FUNCTION "KLASCHKA" : VOID
TITLE =SEQUENZA DOPPIO FOGLIO
AUTHOR : D_T
VERSION : 0.1

BEGIN
NETWORK
TITLE =Pulitura segnale 0 fogli da Klascka
//20131115_Reset o Fogli solo in Ciclo e Posizione di Prelievo
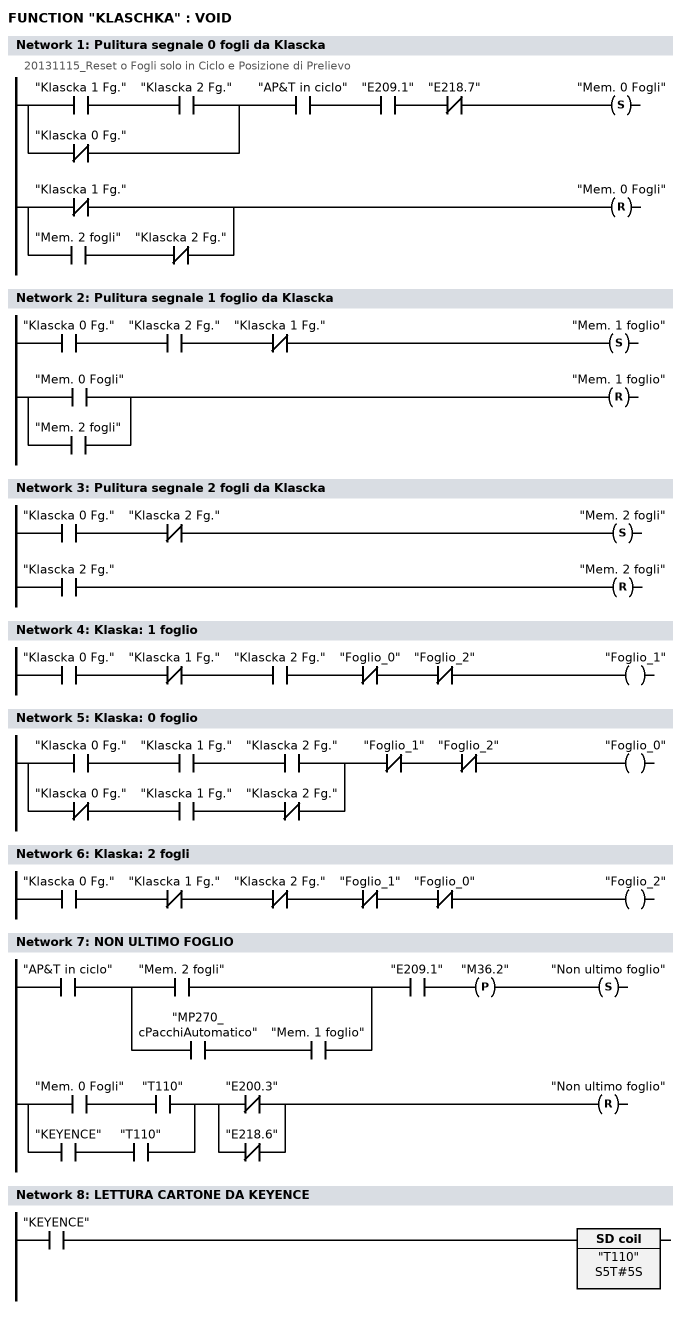
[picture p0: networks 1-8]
      U(    ;
      U     "Klascka 1 Fg.";
      U     "Klascka 2 Fg.";
      ON    "Klascka 0 Fg.";
      )     ;
      U     "AP&T  in ciclo";
      U     "E209.1";
      UN    "E218.7";
      S     "Mem. 0 Fogli";
      U(    ;
      ON    "Klascka 1 Fg.";
      O     ;
      U     "Mem. 2 fogli";
      UN    "Klascka 2 Fg.";
      )     ;
      R     "Mem. 0 Fogli";
      NOP   0;
NETWORK
TITLE =Pulitura segnale 1 foglio da Klascka

      U     "Klascka 0 Fg.";
      U     "Klascka 2 Fg.";
      UN    "Klascka 1 Fg.";
      S     "Mem. 1 foglio";
      U(    ;
      O     "Mem. 0 Fogli";
      O     "Mem. 2 fogli";
      )     ;
      R     "Mem. 1 foglio";
      NOP   0;
NETWORK
TITLE =Pulitura segnale 2 fogli da Klascka

      U     "Klascka 0 Fg.";
      UN    "Klascka 2 Fg.";
      S     "Mem. 2 fogli";
      U     "Klascka 2 Fg.";
      R     "Mem. 2 fogli";
      NOP   0;
NETWORK
TITLE =Klaska: 1 foglio

      U     "Klascka 0 Fg.";
      UN    "Klascka 1 Fg.";
      U     "Klascka 2 Fg.";
      UN    "Foglio_0";
      UN    "Foglio_2";
      =     "Foglio_1";
NETWORK
TITLE =Klaska: 0 foglio

      U(    ;
      U     "Klascka 0 Fg.";
      U     "Klascka 1 Fg.";
      U     "Klascka 2 Fg.";
      O     ;
      UN    "Klascka 0 Fg.";
      U     "Klascka 1 Fg.";
      UN    "Klascka 2 Fg.";
      )     ;
      UN    "Foglio_1";
      UN    "Foglio_2";
      =     "Foglio_0";
NETWORK
TITLE =Klaska: 2 fogli

      U     "Klascka 0 Fg.";
      UN    "Klascka 1 Fg.";
      UN    "Klascka 2 Fg.";
      UN    "Foglio_1";
      UN    "Foglio_0";
      =     "Foglio_2";
NETWORK
TITLE =NON ULTIMO FOGLIO

      U     "AP&T  in ciclo";
      U(    ;
      O     "Mem. 2 fogli";
      O     ;
      U     "MP270_cPacchiAutomatico";
      U     "Mem. 1 foglio";
      )     ;
      U     "E209.1";
      FP    "M36.2";
      S     "Non ultimo foglio";
      U(    ;
      U     "Mem. 0 Fogli";
      U     "T110";
      O     ;
      U     "KEYENCE";
      U     "T110";
      )     ;
      U(    ;
      ON    "E200.3";
      ON    "E218.6";
      )     ;
      R     "Non ultimo foglio";
      NOP   0;
NETWORK
TITLE =LETTURA CARTONE DA KEYENCE

      U     "KEYENCE";
      L     S5T#5S;
      SE    "T110";
      NOP   0;
      NOP   0;
      NOP   0;
      NOP   0;
NETWORK
TITLE =ULTIMO FOGLIO PRELEVATO
//A82.6  VECCHIO SEGNALE ORA NON ESISTE PIU'  PERCHE''?
//MaxZub20101019: T42 da 50MS a 150MS
      U(    ;
      U     "AP&T  in ciclo";
      U     "E209.1";
      U(    ;
      UN    "MP270_cPacchiAutomatico";
      U     "Mem. 1 foglio";
      O     ;
      UN    "Da Comau: Rich.svuotam.";
      UN    "M183.1";
      U     "MP270_cPacchiAutomatico";
      U(    ;
      U     "Mem. 0 Fogli";
      U     "T110";
      O     "T110";
      )     ;
      )     ;
      UN    "Non ultimo foglio";
      L     S5T#500MS;
      SE    "T42";
      NOP   0;
      NOP   0;
      NOP   0;
      U     "T42";
      )     ;
      FP    "One_Shot_ult_foglio";
      S     "Ultimo foglio prelevato";
      U(    ;
      O     "Cambio pacco in corso";
      O     "Non ultimo foglio";
      O(    ;
      U     "E209.1";
      FP    "One_R_Shot_ult_foglio";
      )     ;
      )     ;
      R     "Ultimo foglio prelevato";
      NOP   0;
NETWORK
TITLE =Controllo sequenza lettura klascka OK
//Nel ciclo deve riscontrare la sequenza 2 fogli -> 1 foglio -> 0 fogli
//
      U(    ;
      U     "Mem. 2 fogli";
      S     "Step 1   Klascka";
      U     "E209.1";
      FP    "M37.7";
      R     "Step 1   Klascka";
      U     "Step 1   Klascka";
      )     ;
      UN    "Step 2   Klascka";
      UN    "Step 3   Klascka";
      O     ;
      U(    ;
      U     "Mem. 1 foglio";
      S     "Step 2   Klascka";
      U     "E209.1";
      U     "M37.7";
      R     "Step 2   Klascka";
      U     "Step 2   Klascka";
      )     ;
      U     "Step 1   Klascka";
      UN    "Step 3   Klascka";
      O     ;
      U(    ;
      U     "Mem. 0 Fogli";
      S     "Step 3   Klascka";
      U     "E209.1";
      U     "M37.7";
      R     "Step 3   Klascka";
      U     "Step 3   Klascka";
      )     ;
      U     "Step 1   Klascka";
      U     "Step 2   Klascka";
      O     ;
      UN    "Klascka 0 Fg.";
      UN    "Klascka 1 Fg.";
      UN    "Klascka 2 Fg.";
      =     "Sequenza Klascka OK";
NETWORK
TITLE =Comandi Salita - discesa Klascka

      U     "ON";
      =     L      0.0;
      U     L      0.0;
      U     "Emergenze ripristinate";
      U     "Barriere/ripari ripristi";
      =     L      0.1;
      U     L      0.1;
      U     "Modo man.";
      =     L      0.2;
      U     L      0.2;
      U     "M133.2";
      UN    "M133.3";
      R     "M133.5";
      R     "M133.7";
      S     "M133.4";
      U     L      0.2;
      U     "M133.3";
      UN    "M133.2";
      R     "M133.4";
      R     "M133.6";
      S     "M133.5";
      U     L      0.1;
      U     "Modo auto";
      U     "Cambio produz. in corso";
      =     L      0.2;
      U     L      0.2;
      U(    ;
      O     "Cambio prod.: Passo 7";
      O     "Cambio prod.: Passo 8";
      O     "Cambio prod.: Passo 9";
      )     ;
      R     "M133.7";
      R     "M133.5";
      S     "M133.6";
      U     L      0.2;
      U     "Cambio prod.: Passo 10";
      UN    "E219.0";
      U     "M145.2";
      R     "M133.6";
      R     "M133.4";
      S     "M133.7";
      U     L      0.0;
      U     "E219.0";
      =     L      0.1;
      U     L      0.1;
      U     "M133.5";
      R     "M133.5";
      U     L      0.1;
      U     "M133.7";
      R     "M133.7";
NETWORK
TITLE =Uscite EV salita discesa klascka

      U     "ON";
      =     L      0.0;
      U     L      0.0;
      U(    ;
      U     "M133.4";
      UN    "M133.5";
      O     "M133.6";
      )     ;
      =     "A23.6";
      U(    ;
      U     L      0.0;
      U(    ;
      U     "M133.5";
      UN    "M133.4";
      O     "M133.7";
      )     ;
      UN    "E219.0";
      L     S5T#2S;
      SE    T     62;
      NOP   0;
      NOP   0;
      NOP   0;
      U     T     62;
      )     ;
      L     S5T#200MS;
      SI    "T56";
      NOP   0;
      NOP   0;
      NOP   0;
      U     "T56";
      =     "A23.7";
NETWORK
TITLE =

END_FUNCTION

